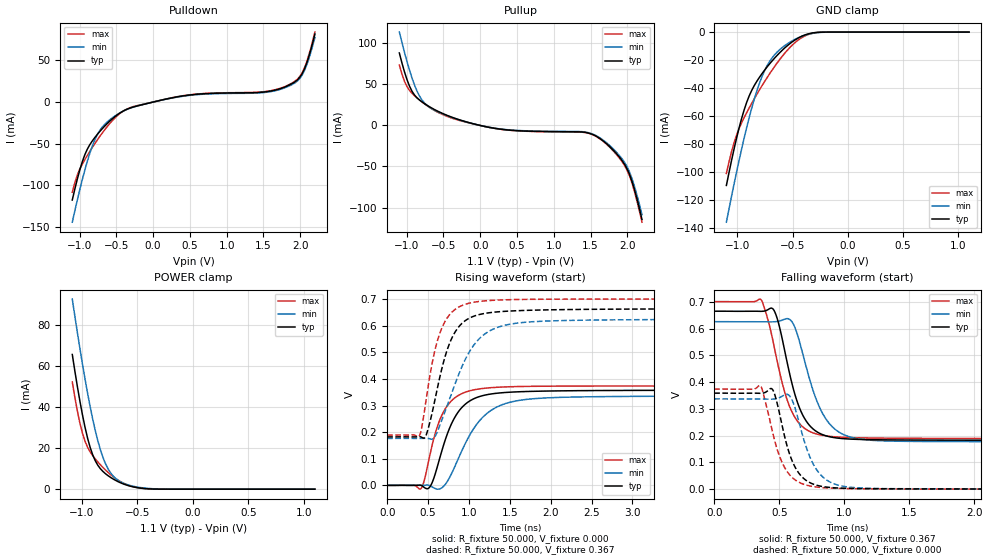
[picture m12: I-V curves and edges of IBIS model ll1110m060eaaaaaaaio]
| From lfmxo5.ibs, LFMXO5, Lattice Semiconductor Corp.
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|   Model ll1110m060eaaaaaaaio
[Model] ll1110m060eaaaaaaaio
| Clamp models do not include dynamic input termination. Please refer to
| the ll1110axxxeaaaaaaain model for input termination.
Model_type I/O
Polarity   Non-Inverting
Enable   Active-Low
Vinl =  0.093V
Vinh =  0.273V
Vmeas =  0.183V
Cref =  30.000pF
Rref =  50.000
Vref =  0.183V
C_comp   5.000pF   4.000pF   5.500pF
[Temperature Range]   25.000   0.125k   -40.000
[Voltage Range]   1.100V   1.050V   1.160V
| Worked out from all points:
|   slope of the pulldown table from 0 to 0.165 V, typ, clamps not added: 49 ohm
|   slope of the pullup table from 0 to 0.165 V, typ, clamps not added: 54.8 ohm
|   GND clamp passes 1 mA (typ) near -0.34 V on its own axis
|   POWER clamp passes 1 mA (typ) near -0.53 V on its own axis
|   rising waveform, R_fixture 50.000, V_fixture 0.000: 20-80 % time 282ps typ, 395ps min, 239ps max; typ from 0 V to 0.358 V
|   rising waveform, R_fixture 50.000, V_fixture 0.367: 20-80 % time 261ps typ, 387ps min, 217ps max; typ from 0.182 V to 0.665 V
|   falling waveform, R_fixture 50.000, V_fixture 0.367: 20-80 % time 159ps typ, 189ps min, 164ps max; typ from 0.665 V to 0.182 V
|   falling waveform, R_fixture 50.000, V_fixture 0.000: 20-80 % time 134ps typ, 153ps min, 141ps max; typ from 0.358 V to 0 V
[GND_clamp]
|Voltage   I(typ)   I(min)   I(max)
-1.1V     -109.7mA   -136mA     -101.1mA
-1.031V   -83.83mA   -108.9mA   -79.25mA
-962mV    -61.81mA   -83.69mA   -64.88mA
-893mV    -45.59mA   -61.04mA   -54.23mA
-824mV    -35.2mA    -42.07mA   -44.52mA
-778mV    -29.85mA   -31.99mA   -38.47mA
-732mV    -25.04mA   -24.18mA   -32.73mA
-663mV    -18.63mA   -16.24mA   -24.64mA
-594mV    -13.03mA   -11.06mA   -17.35mA
-433mV    -3.573mA   -3.549mA   -4.801mA
-272mV    -185.6uA   -413.4uA   -195.8uA
1.1V      0A         0A         0A
[POWER_clamp]
|Voltage   I(typ)   I(min)   I(max)
-1.085V   65.46mA    92.38mA    52.09mA
-1.039V   49.83mA    76.06mA    37.92mA
-993mV    36.02mA    60.7mA     27.13mA
-947mV    24.74mA    46.56mA    20.34mA
-901mV    16.65mA    34.03mA    16.28mA
-855mV    11.62mA    23.53mA    13.22mA
-809mV    8.607mA    15.46mA    10.54mA
-763mV    6.559mA    9.886mA    8.161mA
-694mV    4.241mA    5.164mA    5.156mA
-556mV    1.362mA    1.666mA    1.473mA
-395mV    157uA      339.2uA    107.6uA
1.1V      0A         0A         466pA
[Pulldown]
|Voltage   I(typ)   I(min)   I(max)
-1.1V     -117.9mA   -144.6mA   -108.6mA
-964mV    -71.92mA   -93.46mA   -74.75mA
-828mV    -46.86mA   -53.12mA   -54.68mA
-726mV    -35.44mA   -34.2mA    -41.42mA
-590mV    -22.93mA   -21.33mA   -25.83mA
-318mV    -7.319mA   -7.58mA    -6.947mA
226mV     4.511mA    4.285mA    4.646mA
1.518V    12.17mA    11.56mA    12.54mA
1.824V    19.3mA     18.33mA    19.88mA
2.028V    34.44mA    32.71mA    35.47mA
2.096V    48.95mA    46.51mA    50.42mA
2.2V      81.73mA    77.65mA    84.19mA
[Pullup]
|Voltage   I(typ)   I(min)   I(max)
-1.1V     88.32mA    113.8mA    73.59mA
-996mV    55.91mA    77.94mA    47.28mA
-860mV    33.67mA    41.95mA    33.68mA
-758mV    26.63mA    27.31mA    26.33mA
-622mV    19.41mA    18.58mA    18.27mA
160mV     -2.933mA   -2.787mA   -3.021mA
1.384V    -7.973mA   -7.575mA   -8.213mA
1.622V    -15.55mA   -14.78mA   -16.02mA
1.826V    -31.65mA   -30.06mA   -32.6mA
1.996V    -52.64mA   -50.01mA   -54.22mA
2.098V    -78.11mA   -74.21mA   -80.45mA
2.2V      -114.5mA   -108.8mA   -117.9mA
[Ramp]
| variable   typ   min   max
dV/dt_r   0.215/0.281n   0.202/0.394n   0.224/0.238n
dV/dt_f   0.287/0.224n   0.272/0.270n   0.302/0.225n
R_load = 50.000
[Rising Waveform]
R_fixture = 50.000
V_fixture = 0.000
V_fixture_min = 0.000
V_fixture_max = 0.000
|  time   V(typ)   V(min)   V(max)
0s        3.319uV    89.43uV    -354uV
419ps     -298uV     178.8uV    -9.939mV
534ps     213.6uV    -2.945mV   130mV
665ps     125.9mV    -10.01mV   261.4mV
788ps     232.4mV    44.6mV     318.4mV
929ps     297.7mV    140.6mV    347.1mV
1.136ns   334.6mV    245.1mV    363mV
1.413ns   348.5mV    304mV      369.8mV
3.401ns   357.4mV    335.2mV    373.6mV
30ns      358.4mV    336.9mV    373.6mV
[Rising Waveform]
R_fixture = 50.000
V_fixture = 0.367
V_fixture_min = 0.350
V_fixture_max = 0.386
|  time   V(typ)   V(min)   V(max)
0s        182.2mV    176.5mV    189mV
395ps     182.9mV    176.6mV    186.8mV
472ps     185.5mV    176.9mV    312.9mV
570ps     301.3mV    177.2mV    488.8mV
690ps     464.4mV    263.3mV    606mV
835ps     578.7mV    385.2mV    662.5mV
1.049ns   634.8mV    522.8mV    688mV
1.302ns   651mV      588.2mV    696mV
3.262ns   663.2mV    623.3mV    700.5mV
30ns      664.6mV    625.4mV    700.5mV
[Falling Waveform]
R_fixture = 50.000
V_fixture = 0.367
V_fixture_min = 0.350
V_fixture_max = 0.386
|  time   V(typ)   V(min)   V(max)
0s        664.6mV    625.5mV    700.5mV
363ps     664.2mV    625.1mV    705.7mV
467ps     660.4mV    625.3mV    516.8mV
532ps     539.5mV    633.2mV    379mV
588ps     413.4mV    630.6mV    298.4mV
687ps     270.3mV    493.2mV    229.8mV
820ps     206mV      294.9mV    201.9mV
907ps     193.5mV    232.9mV    196.1mV
1.026ns   187.3mV    197.5mV    192.7mV
30ns      182.2mV    176.5mV    189mV
[Falling Waveform]
R_fixture = 50.000
V_fixture = 0.000
V_fixture_min = 0.000
V_fixture_max = 0.000
|  time   V(typ)   V(min)   V(max)
0s        358.5mV    337mV      373.6mV
355ps     357.9mV    336.5mV    386mV
455ps     366mV      336.3mV    199.7mV
505ps     275.2mV    342.5mV    118.8mV
571ps     143.2mV    351.8mV    58.48mV
648ps     61.06mV    256.7mV    26.38mV
766ps     17.62mV    88.96mV    9.028mV
849ps     8.308mV    39.17mV    4.858mV
976ps     3.5mV      11.9mV     2.254mV
30ns      4.904uV    95.63uV    -354uV
